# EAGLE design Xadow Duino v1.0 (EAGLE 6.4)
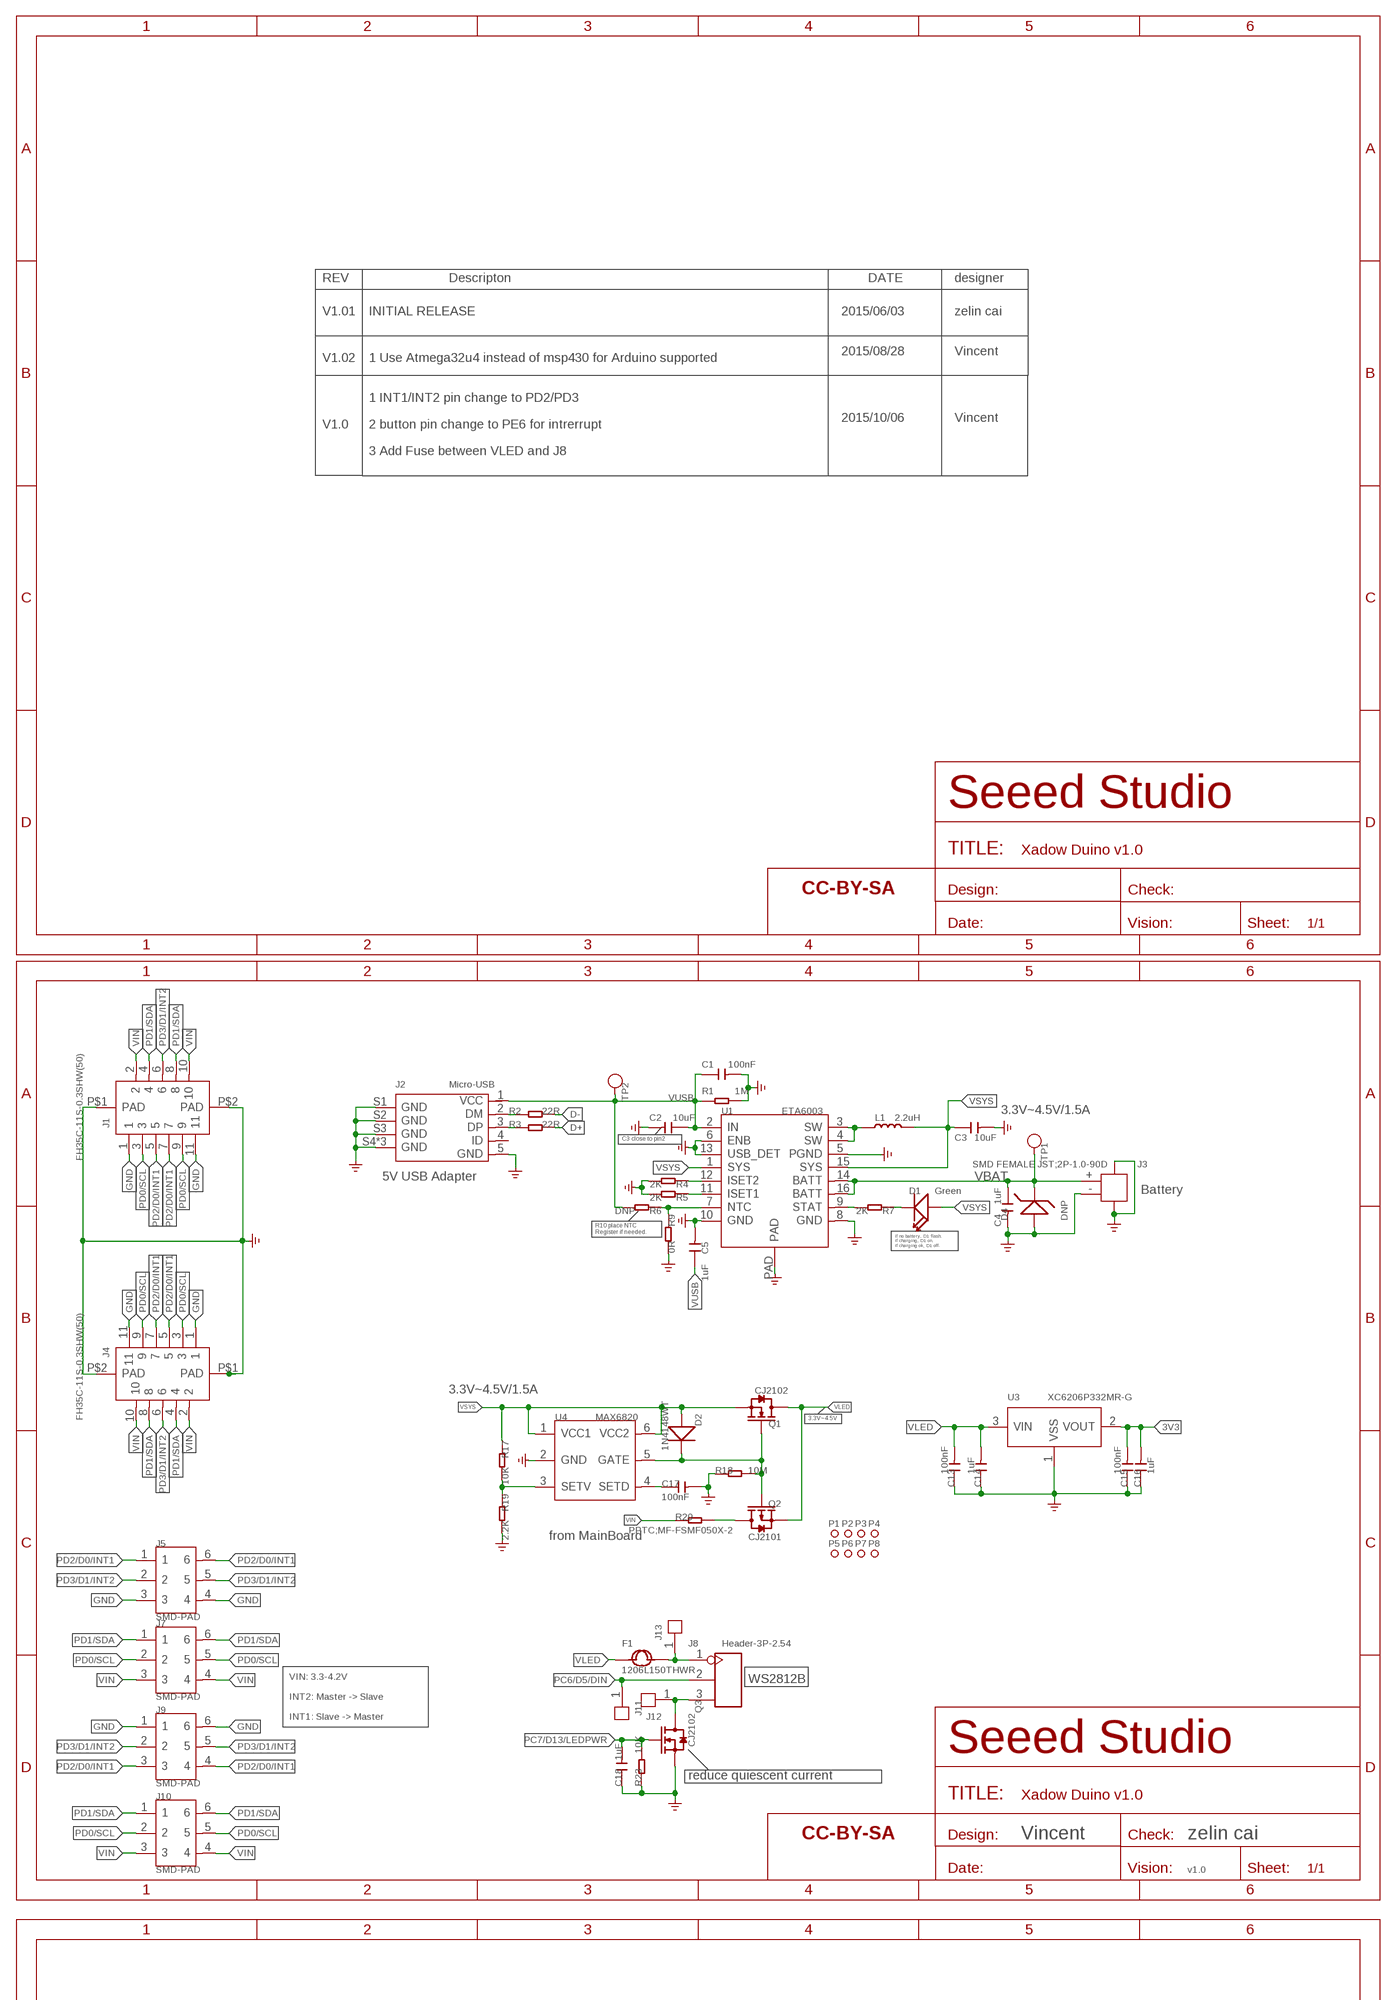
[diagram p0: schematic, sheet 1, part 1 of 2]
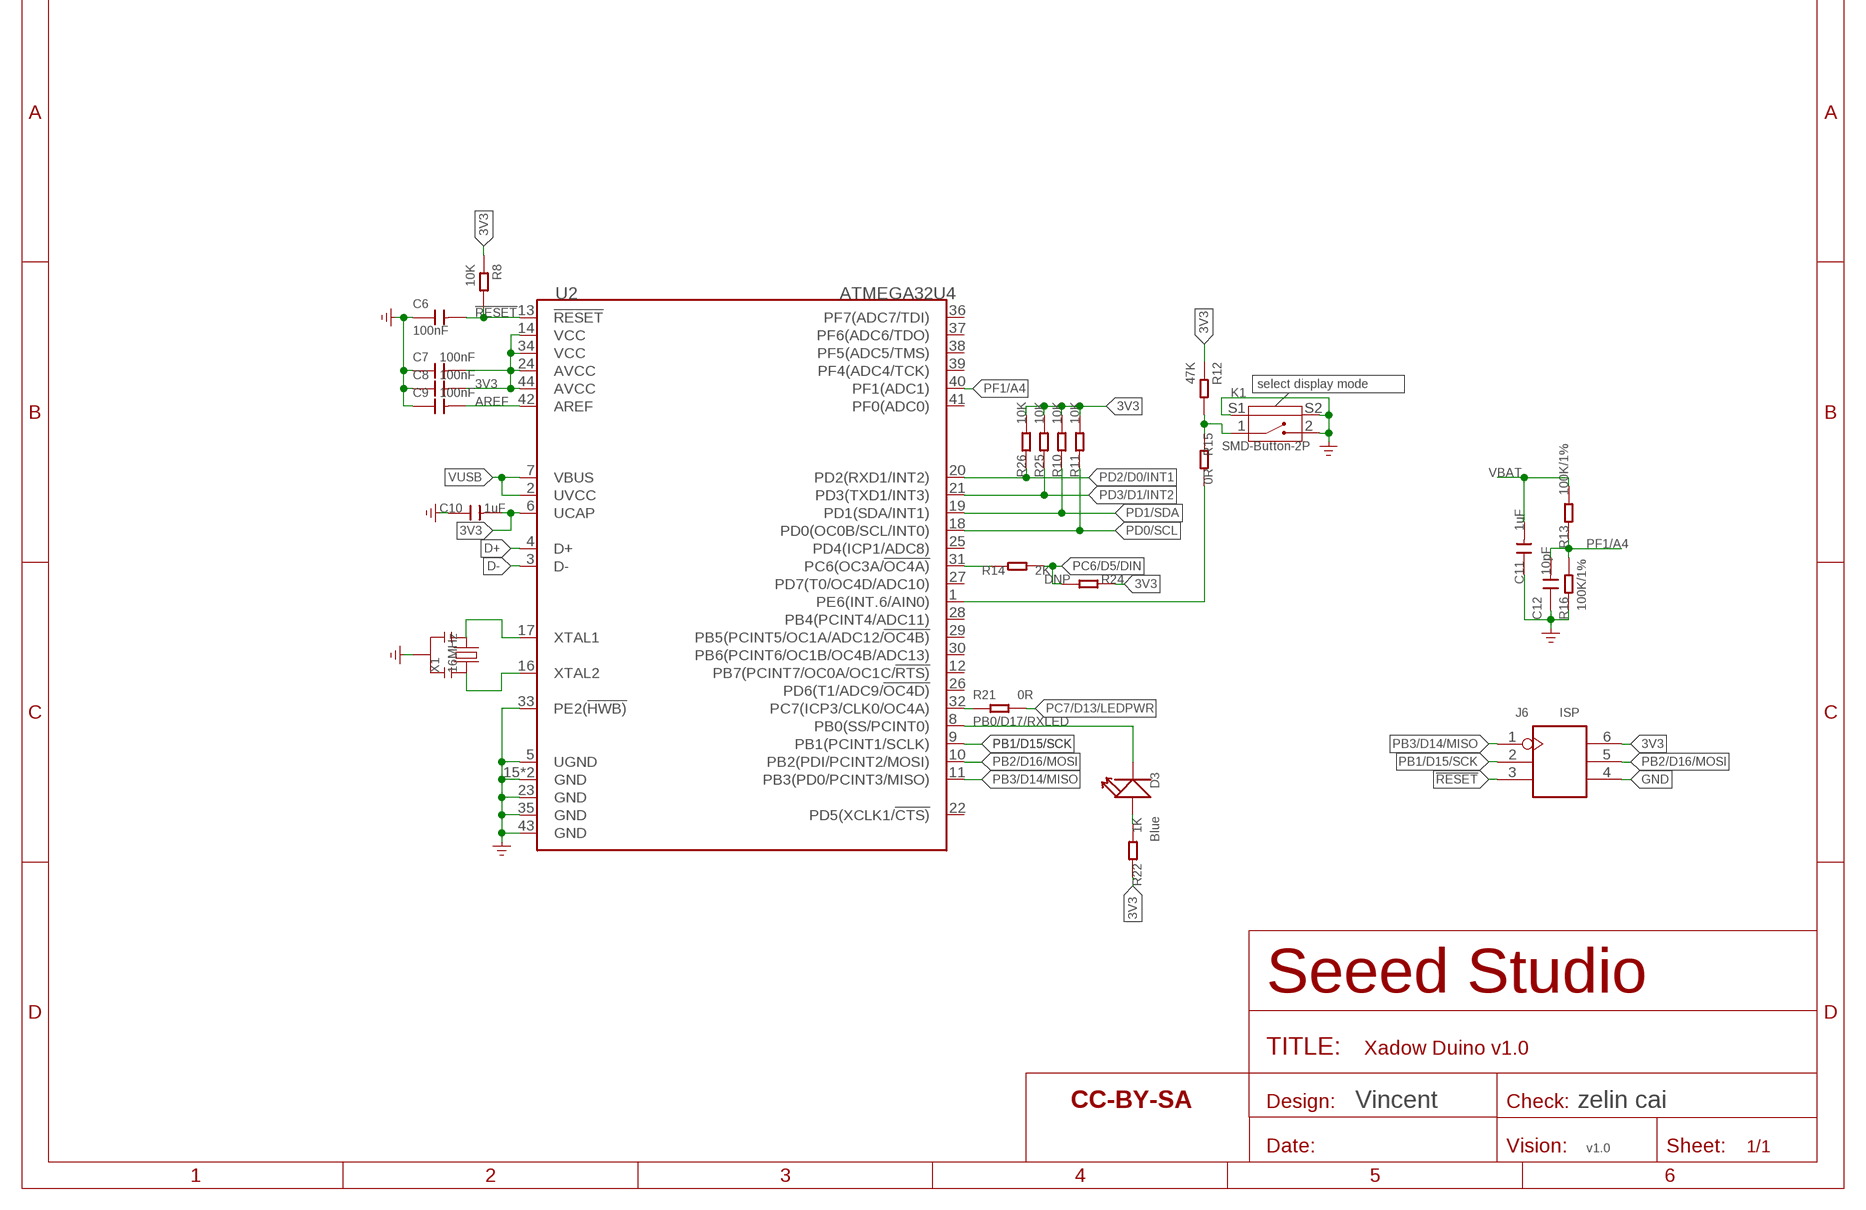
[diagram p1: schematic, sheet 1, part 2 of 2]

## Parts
C1  100nF  CAP-0201  [C0201]
C2  10uF  CAP-0603  [C0603]
C3  10uF  CAP-0603  [C0603]
C4  1uF  CAP-0402  [C0402]
C5  1uF  CAP-0402  [C0402]
C6  100nF  CAP-0201  [C0201]
C7  100nF  CAP-0201  [C0201]
C8  100nF  CAP-0201  [C0201]
C9  100nF  CAP-0201  [C0201]
C10  1uF  CAP-0402  [C0402]
C11  1uF  CAP-0402  [C0402]
C12  10pF  CAP-0201  [C0201]
C13  100nF  CAP-0201  [C0201]
C14  1uF  CAP-0402  [C0402]
C15  100nF  CAP-0201  [C0201]
C16  1uF  CAP-0402  [C0402]
C17  100nF  CAP-0201  [C0201]
C18  1uF  CAP-0402  [C0402]
D1  Green  LED'0402'  [LED-0402]
D2  1N4148WT  DIODE'0603'  [SOD-523]
D3  Blue  LED'0402'  [LED-0402]
D4  DNP  D-ZENER-2P'BZX584CX'  [SOD-523]
F1  1206L150THWR  FUSE'1206'  [F1206]
FR1  SEEEDSTUDIO-OPEN-SCH-FRAME  [SEEEDSTUDIO-PCB-FRAME]
FR2  SEEEDSTUDIO-OPEN-SCH-FRAME  [SEEEDSTUDIO-PCB-FRAME]
FR3  SEEEDSTUDIO-OPEN-SCH-FRAME  [SEEEDSTUDIO-PCB-FRAME]
J1  FH35C-11S-0.3SHW(50)  FPC-CONNECTER-11P(FH35C-11S-0.3SHW(50))  [FPC11-SMD-0.3(FH35C)]
J2  Micro-USB  MICRO-USB5+4P'5+4P'  [MICRO-USB5+4P-SMD-0.65-B]
J3  SMD FEMALE JST;2P-1.0-90D  JST-2P-SMD'1.0'  [HW2-SMD-1.0-90D]
J4  FH35C-11S-0.3SHW(50)  FPC-CONNECTER-11P(FH35C-11S-0.3SHW(50))  [FPC11-SMD-0.3(FH35C)]
J5  SMD-PAD  HEADER6_ROUND  [6P-DIP-2_ROUND]
J6  ISP  HEADER-2X3P-2.54-1.65  [H2X3P-SMD-2.54(1.65)]
J7  SMD-PAD  HEADER6  [6P-DIP-2]
J8  Header-3P-2.54  HEADER-3P-2.0  [H3-2.0]
J9  SMD-PAD  HEADER6_ROUND  [6P-DIP-2_ROUND]
J10  SMD-PAD  HEADER6  [6P-DIP-2]
J11  HEADER-1P-1.5MM  [1P-3.5/1.5MM]
J12  HEADER-1P-1.5MM  [1P-3.5/1.5MM]
J13  HEADER-1P-1.5MM  [1P-3.5/1.5MM]
K1  SMD-Button-2P  BUTTON-2+2P'HQ-TP-1100A'  [SW4-SMD-4.5X3.8X1.8MM-90D]
L1  2.2uH  INDUCTOR/FERRITE-BEAD'0805'  [L0805]
P1  MARK-1.0'ANNULAR'  [ROUND-MARK-1.0]
P2  MARK-1.0'ANNULAR'  [ROUND-MARK-1.0]
P3  MARK-1.0'ANNULAR'  [ROUND-MARK-1.0]
P4  MARK-1.0'ANNULAR'  [ROUND-MARK-1.0]
P5  MARK-1.0'ANNULAR'  [ROUND-MARK-1.0]
P6  MARK-1.0'ANNULAR'  [ROUND-MARK-1.0]
P7  MARK-1.0'ANNULAR'  [ROUND-MARK-1.0]
P8  MARK-1.0'ANNULAR'  [ROUND-MARK-1.0]
Q1  CJ2102  MOSFET-N'SI1304BDL'  [SOT-323]
Q2  CJ2101  MOSFET-P-SOT323  [SOT-323]
Q3  CJ2102  MOSFET-N'SI1304BDL'  [SOT-323]
R1  1M  RES-0201  [R0201]
R2  22R  RES-0201  [R0201]
R3  22R  RES-0201  [R0201]
R4  2K  RES-0201  [R0201]
R5  2K  RES-0201  [R0201]
R6  DNP  RES-0201  [R0201]
R7  2K  RES-0201  [R0201]
R8  10K  RES-0201  [R0201]
R9  0R  RES-0201  [R0201]
R10  10K  RES-0201  [R0201]
R11  10K  RES-0201  [R0201]
R12  47K  RES-0201  [R0201]
R13  100K/1%  RES-0201  [R0201]
R14  2K  RES-0201  [R0201]
R15  0R  RES-0201  [R0201]
R16  100K/1%  RES-0201  [R0201]
R17  10K  RES-0201  [R0201]
R18  10M  RES-0201  [R0201]
R19  2.2K  RES-0201  [R0201]
R20  PPTC;MF-FSMF050X-2  RES-0603  [R0603]
R21  0R  RES-0201  [R0201]
R22  1K  RES-0201  [R0201]
R23  10K  RES-0201  [R0201]
R24  DNP  RES-0201  [R0201]
R25  10K  RES-0201  [R0201]
R26  10K  RES-0201  [R0201]
TP1  TEST-POINT-23  [TP-D23MIL]
TP2  TEST-POINT-23  [TP-D23MIL]
U1  ETA6003  PMIC-ETA6003  [QFN16GA-0.5-3X3MM]
U2  ATMEGA32U4  MCU-ATMEGA32U4-MUR  [QFN44G-0.5-7X7MM]
U3  XC6206P332MR-G  PMIC-XC6206PMR  [SOT-23]
U4  MAX6820  PMIC-MAX6820  [SOT-23-6]
X1  16MHz  CRYSTAL-RESONATOR'SMD'  [3P-SMD-3.6X1.3]

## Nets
3V3: C7.2 C8.2 C10.2 C15.2 C16.2 J6.6 R8.1 R10.2 R11.2 R12.1 R22.1 R24.1 R25.1 R26.2 U2.6(UCAP) U2.14(VCC) U2.24(AVCC) U2.34(VCC) U2.44(AVCC) U3.2(VOUT)
!RESET: C6.2 J6.3 R8.2 U2.13(!RESET)
AREF: C9.2 U2.42(AREF)
D+: R3.2 U2.4(D+)
D-: R2.2 U2.3(D-)
GND: C1.2 C2.2 C3.2 C4.2 C5.2 C6.1 C7.1 C8.1 C9.1 C10.1 C11.1 C12.1 C13.1 C14.1 C15.1 C16.1 C17.2 C18.1 D4.+ J1.1 J1.11 J1.P$1(PAD) J1.P$2(PAD) J2.5(GND) J2.S1(GND) J2.S2(GND) J2.S3(GND) J2.S4(GND) J2.S5(GND) J2.S6(GND) J3.3 J3.4 J3.- J4.1 J4.11 J4.P$1(PAD) J4.P$2(PAD) J5.3 J5.4 J6.4 J9.1 J9.6 K1.2 K1.S1 K1.S2 Q3.2(S) R1.2 R4.2 R5.2 R9.2 R16.1 R18.1 R19.2 R23.1 U1.5(PGND) U1.6(ENB) U1.8(GND) U1.10(GND) U1.13(USB_DET) U1.PAD U2.5(UGND) U2.15(GND) U2.23(GND) U2.33(PE2(!HWB)) U2.35(GND) U2.43(GND) U2.TAB(GND) U3.1(VSS) U4.2(GND) X1.2 ; supply symbol labelled GND_POWER
N$1: Q2.3(D) R20.2
N$2: C17.1 U4.4(SETD)
N$3: D2.- Q1.1(G) Q2.1(G) R18.2 U4.5(GATE)
N$4: R15.2 U2.1(PE6(INT.6/AIN0))
N$5: R7.2 U1.9(STAT)
N$6: L1.1 U1.3(SW) U1.4(SW)
N$7: D1.- R7.1
N$8: R4.1 U1.12(ISET2)
N$9: R5.1 U1.11(ISET1)
N$11: R6.1 R9.1 U1.7(NTC)
N$12: R17.2 R19.1 U4.3(SETV)
N$13: F1.2 J8.1 J13.1
N$14: J8.3 J12.1 Q3.3(D)
N$17: J2.2(DM) R2.1
N$18: J2.3(DP) R3.1
N$19: U2.17(XTAL1) X1.1
N$20: U2.16(XTAL2) X1.3
N$21: R14.1 U2.31(PC6(OC3A/!OC4A))
N$22: R21.1 U2.32(PC7(ICP3/CLK0/OC4A))
N$23: K1.1 R12.2 R15.1
N$24: D3.+ R22.2
PB0/D17/RXLED: D3.- U2.8(PB0(SS/PCINT0))
PB1/D15/SCK: J6.2 U2.9(PB1(PCINT1/SCLK))
PB2/D16/MOSI: J6.5 U2.10(PB2(PDI/PCINT2/MOSI))
PB3/D14/MISO: J6.1 U2.11(PB3(PD0/PCINT3/MISO))
PC6/D5/DIN: J8.2 J11.1 R14.2 R24.2
PC7/D13/LEDPWR: C18.2 Q3.1(G) R21.2 R23.2
PD0/SCL: J1.3 J1.9 J4.3 J4.9 J7.2 J7.5 J10.2 J10.5 R11.1 U2.18(PD0(OC0B/SCL/INT0))
PD1/SDA: J1.4 J1.8 J4.4 J4.8 J7.1 J7.6 J10.1 J10.6 R10.1 U2.19(PD1(SDA/INT1))
PD2/D0/INT1: J1.5 J1.7 J4.5 J4.7 J5.1 J5.6 J9.3 J9.4 R26.1 U2.20(PD2(RXD1/INT2))
PD3/D1/INT2: J1.6 J4.6 J5.2 J5.5 J9.2 J9.5 R25.2 U2.21(PD3(TXD1/INT3))
PF1/A4: C12.2 R13.1 R16.2 U2.40(PF1(ADC1))
VBAT: C4.1 C11.2 D4.- J3.+ R13.2 TP1.T U1.14(BATT) U1.16(BATT)
VIN: J1.2 J1.10 J4.2 J4.10 J7.3 J7.4 J10.3 J10.4 R20.1
VLED: C13.2 C14.2 F1.1 Q1.3(D) Q2.2(S) U3.3(VIN)
VSYS: C3.1 D1.+ D2.+ L1.2 Q1.2(S) R17.1 U1.1(SYS) U1.15(SYS) U4.1(VCC1) U4.6(VCC2)
VUSB: C1.1 C2.1 C5.1 J2.1(VCC) R1.1 R6.2 TP2.T U1.2(IN) U2.2(UVCC) U2.7(VBUS)
Unconnected: J2.4(ID) U2.12(PB7(PCINT7/OC0A/OC1C/!RTS)) U2.22(PD5(XCLK1/!CTS)) U2.25(PD4(ICP1/ADC8)) U2.26(PD6(T1/ADC9/!OC4D)) U2.27(PD7(T0/OC4D/ADC10)) U2.28(PB4(PCINT4/ADC11)) U2.29(PB5(PCINT5/OC1A/ADC12/!OC4B)) U2.30(PB6(PCINT6/OC1B/OC4B/ADC13)) U2.36(PF7(ADC7/TDI)) U2.37(PF6(ADC6/TDO)) U2.38(PF5(ADC5/TMS)) U2.39(PF4(ADC4/TCK)) U2.41(PF0(ADC0))

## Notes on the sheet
- REV | Descripton | DATE | designer
- V1.01 | INITIAL RELEASE | 2015/06/03 | zelin cai
- 2015/08/28 | Vincent
- V1.02 | 1 Use Atmega32u4 instead of msp430 for Arduino supported
- 1 INT1/INT2 pin change to PD2/PD3
- 2015/10/06 | Vincent
- V1.0 | 2 button pin change to PE6 for intrerrupt
- 3 Add Fuse between VLED and J8
- 3.3V~4.5V/1.5A
- C3 close to pin2
- 5V USB Adapter
- Battery
- R10 place NTC 
  Register if needed.
- if no battery, D1 flash.
  if charging, D1 on.
  if charging ok, D1 off.
- 3.3V~4.5V/1.5A
- 3.3V~4.5V
- from MainBoard
- VIN: 3.3-4.2V
- WS2812B
- INT2: Master -> Slave
- INT1: Slave -> Master
- reduce quiescent current
- Vincent | zelin cai
- v1.0
- select display mode
- Vincent | zelin cai
- v1.0

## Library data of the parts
C1-C18 = Discrete-new:CAP: Ceramic Capacitors
D1 D3 = Discrete-new:LED
D2 = Discrete-new:DIODE*
D4 = Discrete-new:D-ZENER-2P: SOD-123:304030008;SOT-23:304030000
F1 = Discrete-new:FUSE
FR1-FR3 = moudle-new:SEEEDSTUDIO-OPEN-SCH-FRAME
J1 J4 = template:FPC-CONNECTER-11P(FH35C-11S-0.3SHW(50))
J2 = Connector-new:MICRO-USB5+4P: 5+4P-SMD-0.65-B:320010000;5+2P-SMD-0.65-AB:340032001
J3 = Connector-new:JST-2P-SMD: 2P-SMD-1.0-90D:320110054;2P-SMD-2.0-90D:320110026
J5 J9 = template:HEADER6_ROUND
J6 = Connector-new:HEADER-2X3P
J7 J10 = template:HEADER6
J8 = Connector-new:HEADER-3P
J11-J13 = Connector-new:HEADER-1P
K1 = Discrete-new:BUTTON-2+2P: SW4-SMD-4.5X3.8X1.8MM-90D:311020035;SW4-SMD-7.0X3.5X3.5MM-90D:311020023
L1 = Discrete-new:INDUCTOR/FERRITE-BEAD
P1-P8 = Discrete-new:MARK-1.0; PARTNO: DNP
Q1 Q3 = Discrete-new:MOSFET-N
Q2 = Discrete-new:MOSFET-P
R1-R26 = Discrete-new:RES
TP1 TP2 = Discrete-new:TEST-POINT
U1 = template:PMIC-ETA6003: 310990023
U2 = IC-new:MCU-ATMEGA32U4: TQFP-44:310010010;VQFN-44:310010016
U3 = IC-new:PMIC-XC6206P: LOW ESR Cap.Compatible Positive Voltage Regulators
U4 = template:PMIC-MAX6820: 310030267
X1 = Discrete:CRYSTAL-RESONATOR: Resonator Small SMD resonator. This is the itty bitty 10/20MHz resonators with built in caps. CSTCE10M0G55 and CSTCE20M0V53. Footprint has been reviewed closely but hasn't been tested yet.

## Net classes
0 default: width 0.025 mm, drill 0.203 mm, clearance 0.102 mm

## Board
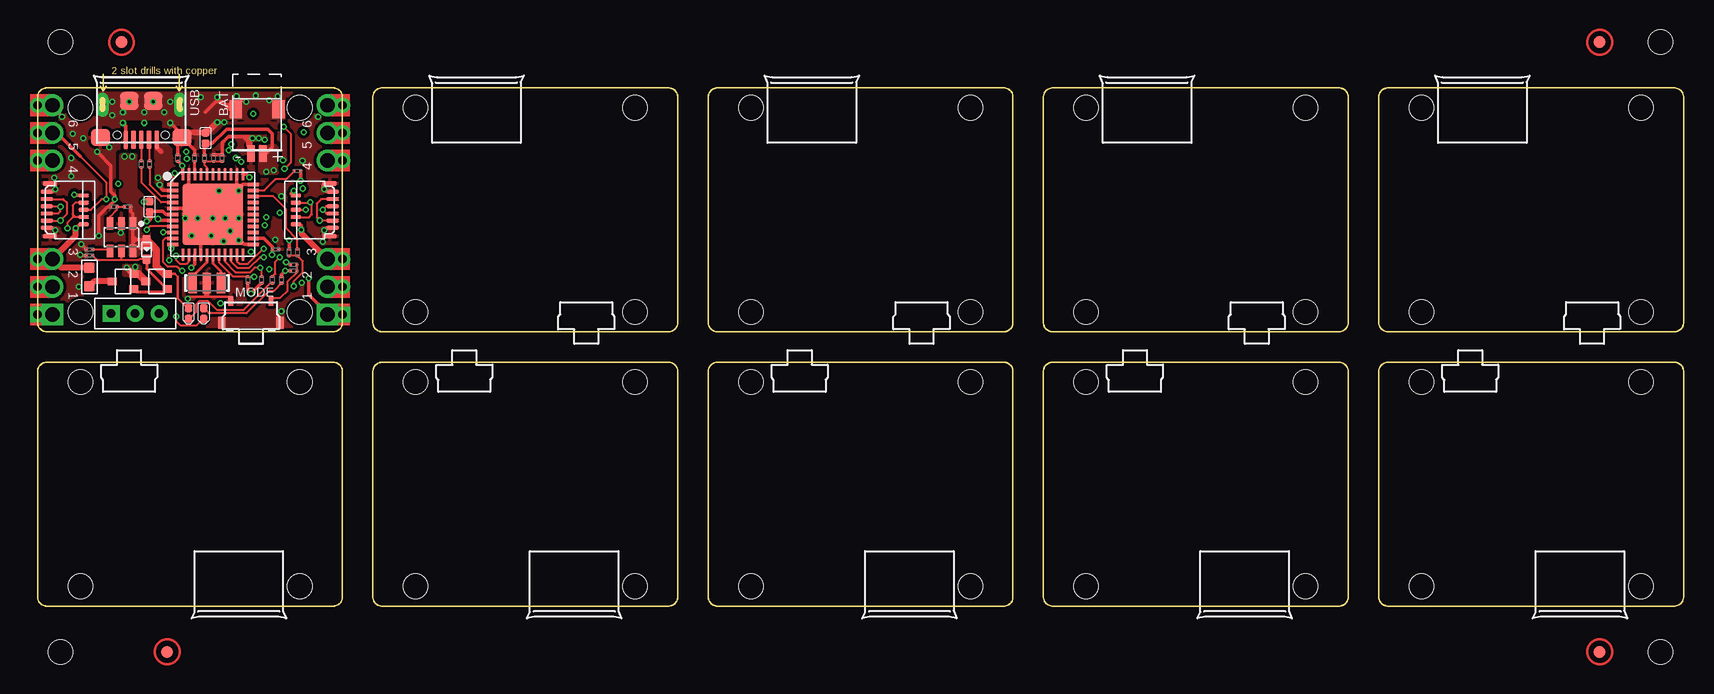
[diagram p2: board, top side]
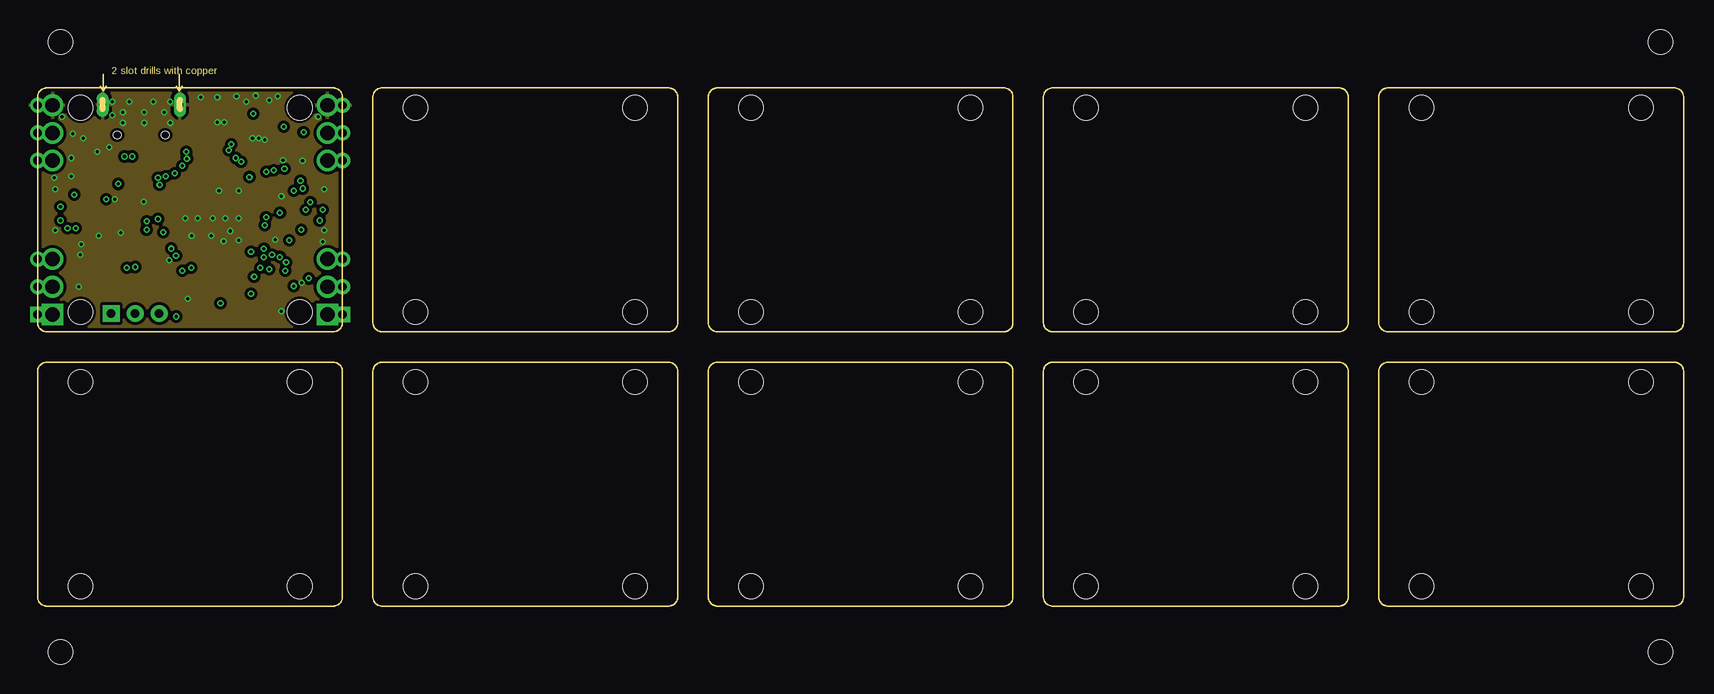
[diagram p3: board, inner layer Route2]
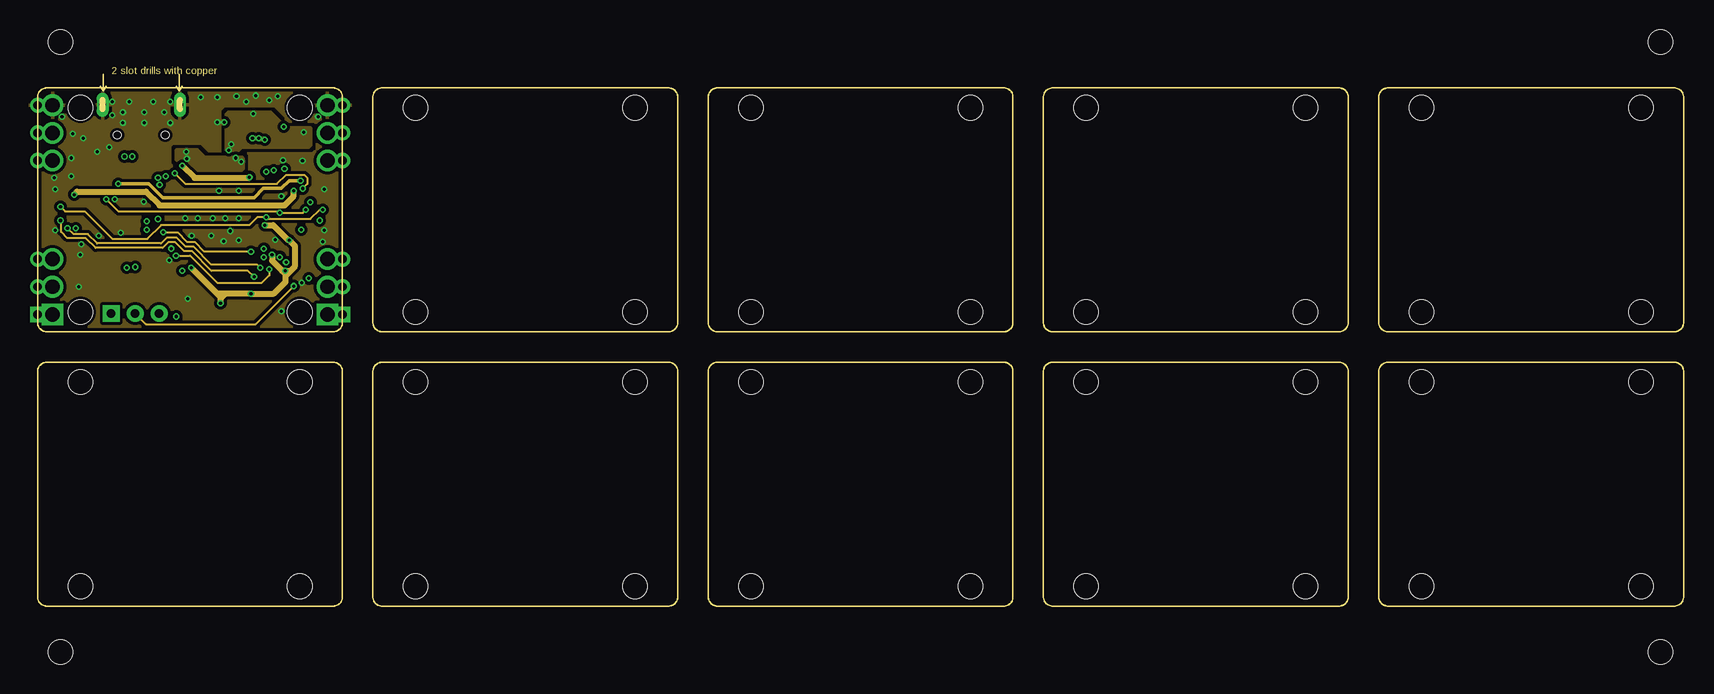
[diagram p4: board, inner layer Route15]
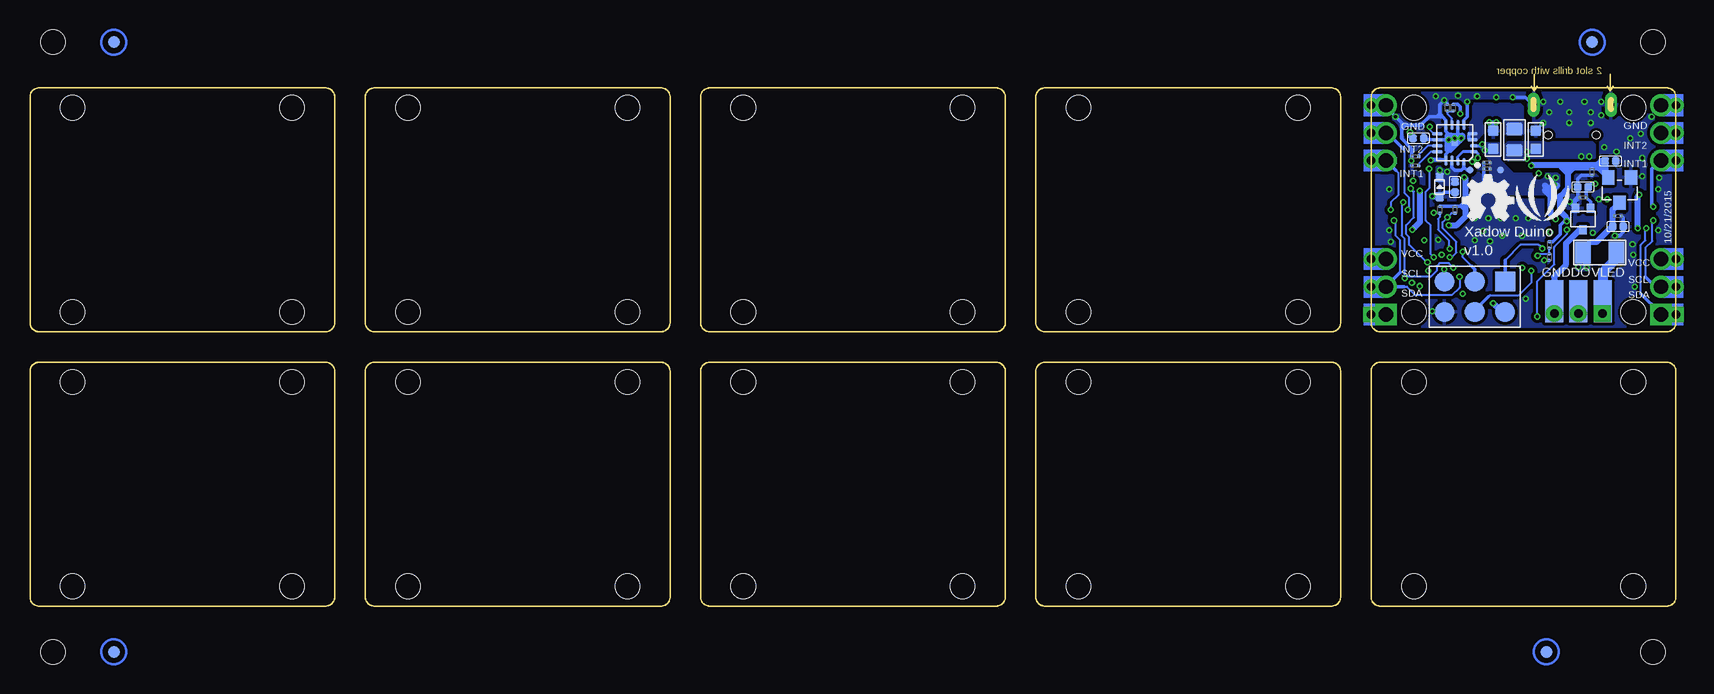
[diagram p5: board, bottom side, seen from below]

Size 137.16 x 43.18 mm. Coordinates in mm from the lower left corner, seen from the top.
Outline: 80 segments
Copper layers (1*2*15*16): Top 0.035mm / dielectric 0.2mm / Route2 0.0175mm / dielectric 0.3mm / Route15 0.0175mm / dielectric 0.2mm / Bottom 0.035mm
Design rules "SeeedStudio_4layer_DRU_no_angle_20140221 *": minimum track width 1mil, minimum drill 10mil, track to track 6mil, track to pad 6mil, pad to pad 6mil, via to via 6mil, smd to smd 0mil, copper to edge 10mil, drill to drill 8mil, minimum pad ring 6mil, minimum via ring 4mil, stop-mask expansion 4mil, vias tented up to drill 100mil, thermal gap 10mil
Holes 2.03 mm at 21.84,24.51 3.56,41.53 21.84,41.53 3.56,24.51 49.78,24.51 31.5,41.53 49.78,41.53 31.5,24.51 77.72,24.51 59.44,41.53 77.72,41.53 59.44,24.51 105.66,24.51 87.38,41.53 105.66,41.53 87.38,24.51 87.38,18.67 105.66,1.65 87.38,1.65 105.66,18.67 59.44,18.67 77.72,1.65 59.44,1.65 77.72,18.67 31.5,18.67 49.78,1.65 31.5,1.65 49.78,18.67 3.56,18.67 21.84,1.65 3.56,1.65 21.84,18.67 133.6,24.51 115.32,41.53 133.6,41.53 115.32,24.51 115.32,18.67 133.6,1.65 115.32,1.65 133.6,18.67 1.9,46.99 135.26,46.99 135.26,-3.81 1.9,-3.81
bRestrict: 1 lines

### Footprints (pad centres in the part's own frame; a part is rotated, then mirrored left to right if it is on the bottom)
C0201 = smd 0.279 x 0.318: 1 -0.279,0; 2 0.279,0
C0603 = smd 0.889 x 0.889: 1 0,0.762; 2 0,-0.762
C0402 = smd 0.635 x 0.635: 1 0,0.445; 2 0,-0.445
LED-0402 = smd 0.635 x 0.635: + -0.445,0; - 0.445,0
SOD-523 = smd 0.762 x 0.7: + -0.8,0; - 0.8,0
F1206 = smd 1.27 x 1.778: 1 -1.397,0; 2 1.397,0
FPC11-SMD-0.3(FH35C) = smd 0.3 x 1: 1 -1.5,-3.075; 3 -0.9,-3.075; 5 -0.3,-3.075; 7 0.3,-3.075; 9 0.9,-3.075; 11 1.5,-3.075 | smd 0.3 x 0.85: 2 -1.2,0; 4 -0.6,0; 6 0,0; 8 0.6,0; 10 1.2,0 | smd 0.4 x 1.15: P$1 2.2,-2.8; P$2 -2.2,-2.8
MICRO-USB5+4P-SMD-0.65-B = smd 0.381 x 1.524: 1 -1.3,-0.25; 2 -0.65,-0.25; 3 0,-0.25; 4 0.65,-0.25; 5 1.3,-0.25 | smd 1.6 x 1.397: S1 -3.4,-0.427; S6 3.4,-0.427 | drill 0.508 pad 1.016 long: S2 -3.226,-3.175; S5 3.226,-3.175 | smd 1.5 x 1.5: S3 -1,-3.5; S4 1,-3.5 | hole 0.635: -2,-0.65; 2,-0.65
HW2-SMD-1.0-90D = smd 1.524 x 1.016: 3 -3.429,1.778; 4 -3.429,-1.778 | smd 1.397 x 0.635: + 0.254,0.508; - 0.254,-0.508
6P-DIP-2_ROUND = drill 0.7 pad 1.27: 1 -2.3,0; 2 0,0; 3 2.3,0 | drill 1.2 pad 1.8: 4 2.3,1.25; 5 0,1.25; 6 -2.3,1.25
H2X3P-SMD-2.54(1.65) = smd 1.65 x 1.65: 1 -1.27,2.54; 2 -1.27,0; 3 -1.27,-2.54; 4 1.27,-2.54; 5 1.27,0; 6 1.27,2.54
6P-DIP-2 = drill 0.7 pad 1.27 square: 1 -2.3,0 | drill 0.7 pad 1.27: 2 0,0; 3 2.3,0 | drill 1.2 pad 1.8: 4 2.3,1.25; 5 0,1.25 | drill 1.2 pad 1.8 square: 6 -2.3,1.25
H3-2.0 = drill 0.7 pad 1.4 square: 1 0,2 | drill 0.7 pad 1.4: 2 0,0; 3 0,-2
1P-3.5/1.5MM = smd 1.5 x 3.5: 1 0,0
SW4-SMD-4.5X3.8X1.8MM-90D = smd 0.4 x 0.8: 1 -1.675,-1.277; 2 1.675,-1.277 | smd 0.6 x 1: S1 -2.425,0.5; S2 2.425,0.5
L0805 = smd 1.016 x 1.397: 1 -0.889,0; 2 0.889,0
ROUND-MARK-1.0 = smd 1.016 x 1.016: P$1 0,0
SOT-323 = smd 0.635 x 0.762: 1 -0.635,-0.889; 2 0.635,-0.889; 3 0,0.889
R0201 = smd 0.279 x 0.318: 1 -0.279,0; 2 0.279,0
R0603 = smd 0.889 x 0.889: 1 0,0.762; 2 0,-0.762
TP-D23MIL = smd 0.6 x 0.6: T 0,0
QFN16GA-0.5-3X3MM = smd 0.65 x 0.28: 1 -1.575,0.75; 2 -1.575,0.25 | smd 0.85 x 0.28: 3 -1.475,-0.25; 4 -1.475,-0.75; 9 1.475,-0.75; 10 1.475,-0.25; 11 1.475,0.25; 12 1.475,0.75 | smd 0.28 x 0.85: 5 -0.75,-1.475; 6 -0.25,-1.475; 7 0.25,-1.475; 8 0.75,-1.475; 13 0.75,1.475; 14 0.25,1.475 | smd 0.28 x 0.65: 15 -0.25,1.575; 16 -0.75,1.575 | smd 0.508 x 0.508: PAD 0,0
QFN44G-0.5-7X7MM = smd 1 x 0.3: 1 -3.35,2.5; 2 -3.35,2; 3 -3.35,1.5; 4 -3.35,1; 5 -3.35,0.5; 6 -3.35,0; 7 -3.35,-0.5; 8 -3.35,-1; 9 -3.35,-1.5; 10 -3.35,-2; 11 -3.35,-2.5; 23 3.35,-2.5; 24 3.35,-2; 25 3.35,-1.5; 26 3.35,-1; 27 3.35,-0.5; 28 3.35,0; 29 3.35,0.5; 30 3.35,1; 31 3.35,1.5; 32 3.35,2; 33 3.35,2.5 | smd 0.3 x 1: 12 -2.5,-3.35; 13 -2,-3.35; 14 -1.5,-3.35; 15 -1,-3.35; 16 -0.5,-3.35; 17 0,-3.35; 18 0.5,-3.35; 19 1,-3.35; 20 1.5,-3.35; 21 2,-3.35; 22 2.5,-3.35; 34 2.5,3.35; 35 2,3.35; 36 1.5,3.35; 37 1,3.35; 38 0.5,3.35; 39 0,3.35; 40 -0.5,3.35; 41 -1,3.35; 42 -1.5,3.35; 43 -2,3.35; 44 -2.5,3.35 | smd 5.08 x 5.08: TAB 0,0
SOT-23 = smd 1.016 x 1.2: 1 -0.95,-1.06; 2 0.95,-1.06; 3 0,1.06
SOT-23-6 = smd 0.55 x 1.016: 1 -0.95,-1.143; 2 0,-1.143; 3 0.95,-1.143; 4 0.95,1.143; 5 0,1.143; 6 -0.95,1.143
3P-SMD-3.6X1.3 = smd 0.7 x 1.7: 1 -1.2,0; 2 0,0; 3 1.2,0

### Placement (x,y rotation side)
C1  15.75,36.96 180 bottom
C2  15.24,38.86 180 bottom
C3  11.68,38.86 180 bottom
C4  18.42,34.92 0 bottom
C5  21.46,38.99 90 bottom
C6  10.54,29.08 90 bottom
C7  19.81,29.72 180 top
C8  11.68,37.34 270 top
C9  13.08,37.34 270 top
C10  9.33,33.27 0 top
C11  13.99,39 0 top
C12  14.67,37.34 270 top
C13  4.83,32.51 180 bottom
C14  4.83,31.62 270 bottom
C15  6.99,36.2 90 bottom
C16  5.46,37.08 270 bottom
C17  4.32,29.72 180 top
C18  7.75,34.92 90 bottom
D1  12.57,24.38 270 top
D2  9.08,29.72 270 top
D3  13.84,24.38 270 top
D4  19.68,34.92 90 bottom
F1  6.35,29.46 0 bottom
FR1  not placed on the board
FR2  not placed on the board
FR3  not placed on the board
J1  21.53,33.02 90 top
J2  8.64,38.61 180 top
J3  18.29,37.97 270 top
J4  3.84,33.02 270 top
J5  25.4,39.43 90 top
J6  16.76,25.78 270 bottom
J7  25.4,26.61 90 top
J8  8.13,24.38 90 top
J9  0,39.43 270 top
J10  0,26.61 90 bottom
J11  8.13,25.4 0 bottom
J12  10.16,25.4 0 bottom
J13  6.1,25.4 0 bottom
K1  17.78,24.13 180 top
L1  13.46,38.86 270 bottom
P1  not placed on the board
P2  not placed on the board
P3  not placed on the board
P4  not placed on the board
P5  not placed on the board
P6  not placed on the board
P7  not placed on the board
P8  not placed on the board
Q1  9.91,27.05 90 top
Q2  7.11,27.05 90 top
Q3  7.75,32.26 180 bottom
R1  15.75,36.45 180 bottom
R2  9.33,36.83 270 top
R3  8.64,36.83 270 top
R4  21.72,36.7 180 bottom
R5  21.72,37.47 180 bottom
R6  18.55,41.53 90 bottom
R7  19.56,27.18 90 top
R8  10.54,30.1 270 bottom
R9  19.05,41.53 90 bottom
R10  18.67,27.18 270 top
R11  17.53,27.18 270 top
R12  21.34,27.94 0 top
R13  13.91,37.34 90 top
R14  21.65,29.46 270 top
R15  21.34,28.45 180 top
R16  15.37,37.34 270 top
R17  7.49,33.27 180 top
R18  4.32,29.21 0 top
R19  6.35,33.27 180 top
R20  4.32,27.43 0 top
R21  21.65,36.26 0 top
R22  20.32,27.18 270 top
R23  7.75,34.04 0 bottom
R24  20.96,29.46 270 top
R25  19.68,33.02 270 bottom
R26  18.42,33.02 90 bottom
TP1  17.14,36.32 0 bottom
TP2  14.61,36.32 0 bottom
U1  18.42,38.61 180 bottom
U2  14.61,32.64 0 top
U3  4.7,34.67 180 bottom
U4  6.99,30.73 180 top
U$1  [OSHW_FILLX150_NOTEXT]  17.78,32.13 0 bottom
U$3  [SEEED-LOGO-150]  13.33,32.13 0 bottom
X1  14.1,26.92 180 top

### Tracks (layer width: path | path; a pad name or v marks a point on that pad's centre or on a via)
3V3  (via drill 0.25 pad 0.51)
  Top 0.254: C8.2 11.71,37.06
  Top 0.305: C10.2 9.4,32.89 10.41,32.89 10.67,32.64 U2.6 | U2.14 13.11,28.5 v12.8,28.19 | U2.34 17.41,35.99 v17.65,35.75 | U2.44 12.11,36.66 v12.07,36.7 11.71,37.06 | U2.24 18.85,30.64 19.53,29.96 C7.2 v19.53,29.29 | R11.2 17.53,26.29 v17.78,26.04 18.64,26.9 R10.2 | R22.1 20.32,27.62 v20.64,27.94 R12.1 | R24.1 20.96,30.48 v20.96,30.49
  Top 0.508: C10.2 9.33,32.32 v9.09,32.08
  Route15 0.305: v20.96,30.49 20.96,30.47 21.21,30.23
  Route15 0.508: v12.07,36.7 13.08,35.69 17.59,35.69 v17.65,35.75 | 15.62,26.04 v17.78,26.04 19.68,26.04 20.64,26.99 20.64,27.5 | 15.62,26.04 15.24,26.04 | 15.24,26.04 14.96,26.04 | 14.96,26.04 v12.8,28.19 | v15.24,25.23 15.24,25.65 | 15.24,25.76 15.24,26.04 | 15.24,25.65 15.24,25.76 | 15.24,25.76 14.96,26.04 | 15.24,25.65 15.62,26.04 | v19.53,29.29 19.53,28.79 20.38,27.94 | v20.64,27.94 20.38,27.94 | v20.64,27.94 20.64,27.5 | v20.64,27.94 21.08,27.94 | 21.08,27.94 21.46,28.32 21.46,29.99 v20.96,30.49 20.88,30.49 19.63,31.74 v18.92,31.74 | 20.64,27.5 21.08,27.94 | 20.38,27.94 20.7,27.62
  Bottom 0.305: R8.1 10.26,30.38 9.65,30.99 9.65,31.75 9.32,32.08 9.14,32.08 | 9.08,32.07 v9.09,32.08 9.14,32.08 | 8.99,32.23 9.14,32.08 | 9.02,32 9.14,32.13 | C15.2 6.83,36.47 6.73,36.58 | 18.01,33.3 R26.2 R25.1 | 17.93,33.3 17.55,33.3 17.53,33.27 | 18.01,33.3 17.65,33.66 | 18.01,33.3 17.93,33.3 | 17.93,33.3 17.65,33.02
  Bottom 0.508: v17.65,35.75 17.53,35.62 17.53,33.27 17.53,32.47 18.26,31.74 v18.92,31.74 | 9.02,36.58 9.02,36.07 | 9.02,36.07 9.02,34.8 9.65,34.16 9.65,32.89 9.14,32.38 9.14,32.13 9.14,32.08 | J6.6 14.52,24.51 v15.24,25.23 | 6.48,36.83 6.22,37.08 C16.2 5.91,35.86 5.78,35.86 U3.2 | 6.54,36.77 6.73,36.58 | 6.48,36.83 6.41,36.77 | 6.41,36.77 5.97,36.32 | 6.48,36.58 6.1,36.58 | 9.02,36.58 9.53,36.58 9.02,36.07 | 9.02,36.58 8.51,36.58 | 8.51,36.58 6.73,36.58 | 9.02,36.07 8.51,36.58 | 6.73,36.58 6.48,36.58 | 6.48,36.58 5.97,36.07 | 6.48,36.7 6.41,36.77 | v12.07,36.7 12,36.77 6.54,36.77 | 6.54,36.77 6.48,36.83
!RESET  (via drill 0.25 pad 0.51)
  Top 0.152: U2.13 12.61,28.72 12.39,28.5 11.89,28.5 11.53,28.85 v11.53,29.2
  Route15 0.152: v11.53,29.2 12.71,29.2 14.99,26.92 18.67,26.92 19.3,27.56 v19.3,28.07
  Bottom 0.152: v11.53,29.21 v11.53,29.2 11.42,29.31 10.67,29.31 10.62,29.36 C6.2 R8.2 | 19.3,27.81 v19.3,28.07
  Bottom 0.305: J6.3 19.3,27.81
AREF
  Top 0.254: U2.42 13.11,37.03 C9.2
D+
  Top 0.152: U2.4 10.3,33.64 8.64,35.31 R3.2
D-
  Top 0.152: R2.2 9.33,35.12 10.31,34.14 U2.3
GND  (via drill 0.25 pad 0.51)
  Top 0.203: X1.2 14.1,26.04 | 14.1,26.04 14.22,25.91 | 14.22,25.91 14.35,25.78 | 14.35,25.78 15.87,25.78 16.11,25.55 K1.2 | 14.35,25.78 12.69,25.78 v12.52,25.62 | 14.1,26.04 13.97,25.91 | 13.97,25.91 13.87,25.81 14,25.81 14.1,25.91 | 13.97,25.91 13.97,26.29 | 14.22,25.91 14.22,26.29
  Top 0.305: U2.5 12.07,33.14 12.32,32.89 v12.32,32.32 12.32,31.38 v12.83,30.87 | J4.P$1 1.29,30.82 1.52,31.05 1.52,31.24 v1.46,31.3 1.25,31.52 J4.11 | J4.1 1.25,34.52 v1.46,34.73 1.52,34.8 1.52,34.99 1.29,35.22 J4.P$2 | J9.6 1.25,41.55 v2.03,40.77 | J1.P$2 24.04,30.82 23.81,31.05 23.81,31.24 v23.88,31.3 24.09,31.52 J1.1 | J1.11 24.09,34.52 v23.88,34.73 23.75,34.86 23.75,35.05 23.92,35.22 J1.P$1 | J3.3 19.81,41.4 | 16.51,41.66 J3.4 16,41.4 15.75,41.66 | 16.51,41.66 17.02,42.16 17.27,42.16 v17.4,42.04 | 15.75,41.66 15.62,41.78 | J2.S1 12.04,39.27 v11.05,40.26 | 12.07,39 13.08,37.99 C9.1 | 12.07,39 J2.S1 | U2.33 17.11,35.14 16.76,34.8 v16.76,34.61 16.73,34.64 16.61,34.64 U2.35 | U2.TAB v14.61,32.32 | U2.23 17.23,30.14 16.45,30.92 14.48,30.92 | U2.15 13.61,30.24 14.29,30.92 14.48,30.92 | U2.43 12.61,34.77 12.95,34.42 14.92,34.42 v15.11,34.61 | 17.65,39.12 15.87,39.12 15.37,38.61 R16.1 C12.1 | 17.65,39.12 17.78,39.12 v17.91,38.99 17.78,38.86 J3.- 17.78,38.1 17.53,38.35 17.53,38.73 | 17.53,38.73 17.53,38.99 17.65,39.12 | 17.53,38.73 17.27,38.99 | 12.14,39.14 J2.S1 | 15.75,41.66 16.51,41.66 | 15.62,41.78 15.95,41.78 | 15.95,41.78 16.51,41.78 | 15.95,41.78 16.15,41.99 | 13.97,41.15 14.86,42.04 | 15.62,41.78 15.37,42.04 15.24,42.04 | 14.86,42.04 15.24,42.04 | 14.86,42.04 14.99,42.16 v14.99,42.42 14.99,42.29 15.24,42.04 | C8.1 11.68,38.61 12,38.93 12.07,39 | U4.2 6.99,31.18 v6.92,31.12 | J2.5 7.34,40.03 v7.11,40.26 | C17.2 4.04,29.74 v3.62,30.16 | R18.1 3.62,29.21 v3.56,29.27 | 14.48,30.92 v14.48,30.87 | v5.08,30.86 5.08,32.51 5.84,33.27 R19.2 6.07,33.44 6.41,33.78 v6.41,33.91 6.41,34.23 6.1,34.54 6.1,36.7 v4.95,37.85
  Top 0.508: C10.1 8.86,33.72 v8.84,33.69 | 12,38.93 12.52,39.44 C11.1 14.11,39.44 v14.99,40.32
  Bottom 0.254: U1.10 20.89,38.86 C5.2
  Bottom 0.305: U1.10 18.55,38.86 v18.42,38.99 | 19.43,40.77 19.17,40.5 U1.8 19.17,39.55 18.92,39.31 18.73,39.31 v18.42,38.99 | 19.43,40.77 19.68,41.02 | C3.2 v11.05,40.26 | J5.4 24.15,41.55 v23.37,40.77 22.86,40.26 | 18.86,39.05 18.86,37.97 19.17,37.67 U1.13 19.24,37.21 20.38,37.21 v20.45,37.15 | R1.2 C1.2 16.03,35.39 | C4.2 19.33,34.48 D4.+ | C6.1 10.97,28.8 v10.99,28.82 | U1.6 18.17,39.45 | 18.17,39.45 18.17,39.24 v18.42,38.99 | 18.14,39.42 18.17,39.45 | 22.73,40.13 22.76,40.16 | 22.76,40.16 22.86,40.26 | 19.68,41.02 19.68,41.78 v19.3,42.16 19.05,41.91 R9.2 | U1.5 17.67,40.5 17.4,40.77 v17.4,42.04 | R5.2 22,38.06 22.86,38.93 22.86,39.75 | R4.2 22,37.03 v22.07,37.11 | v15.56,40.32 v14.99,40.32 15.24,40.07 C2.2 15.24,40 15.49,40.26 | 15.49,40.26 v15.56,40.32 | v15.56,40.32 15.62,40.26 15.49,40.26 | v13.59,42.42 12.57,42.42 11.94,41.78 | R23.1 8.19,34.2 C18.1 8.19,35.62 7.9,35.92 C15.1 | 8.89,33.66 Q3.2 8.38,33.68 R23.1 | v5.08,30.86 4.7,30.86 4.38,31.18 C14.1 4.38,32.35 C13.1 | R23.1 8.25,34.04 8.64,33.66 8.8,33.66 v8.84,33.69 | 19.94,40.77 20.57,40.77 21.27,40.07 22.54,40.07 | 19.94,40.77 19.43,40.77 | 22.86,39.75 22.86,40.26 | 19.68,41.02 19.94,40.77 | 22.54,40.07 22.73,40.07 22.8,40.13 22.76,40.16 | 22.54,40.07 22.86,39.75
  Bottom 0.508: D4.+ 20.28,34.12 v20.32,34.16
  other vias: 5.97,38.23 7.62,42.04 9.65,42.04 11.05,42.04 6.22,42.04 20.32,24.57 16.76,32.32 19.81,30.54 22,26.94 23.77,30.37 3.81,38.99 2.79,35.81 8.89,40.26 1.4,35.69 3.43,26.61 18.92,38.86 16.57,42.48 20,42.48 16.07,31.25 16.76,30.49 7.11,41.15 8.89,41.15 10.54,41.15 18.16,42.55 6.22,40.89 2.92,39.37 2.79,37.34 13.33,32.32 15.62,32.32 15.49,30.42
  pour Top (isolate 0.254, rank 6): -0.64,43.81 26.04,43.81 26.04,22.22 -0.64,22.22
  pour Route2 (isolate 0.254, rank 6): -0.64,43.81 26.04,43.81 26.04,22.22 -0.64,22.22
  pour Route15 (isolate 0.254, rank 6): -0.64,43.81 26.04,43.81 26.04,22.22 -0.64,22.22
  pour Bottom (isolate 0.254, rank 6): -0.64,43.81 26.04,43.81 26.04,22.22 -0.64,22.22
  pour Top (isolate 0.254, no thermals): 14.48,22.86 14.48,24.64 20.57,24.64 20.57,22.86
  pour Top (isolate 0.254, no thermals): 4.95,40.64 20.57,40.64 20.57,43.05 4.95,43.05
N$1
  Top 0.508: Q2.3 4.7,27.05 R20.2
N$2
  Top 0.152: C17.1 5.91,29.72 U4.4
N$3
  Top 0.152: D2.- 8.47,28.92 8.38,28.83 7.11,28.83 | R18.2 4.98,28.83 6.86,28.83 | 7.11,28.83 6.99,28.83 | 6.99,28.83 6.86,28.83 | U4.5 6.99,28.96 | 6.99,28.96 6.99,28.83 | 6.99,28.96 6.86,28.83 | 6.99,28.96 7.11,28.83
  Top 0.254: Q1.1 10.67,26.42 | 10.67,26.42 10.41,26.16 8.25,26.16 Q2.1 | 10.67,26.42 10.67,26.54 9.08,28.13 D2.-
N$4  (via drill 0.25 pad 0.51)
  Top 0.152: U2.1 11.26,35.89 v11.43,36.07 | R15.2 20.89,28.45 v20.7,28.64
  Route15 0.152: v11.43,36.07 12.32,35.18 19.94,35.18 20.7,35.94 22.22,35.94 22.48,35.69 22.48,35.18 v22.1,34.8
  Bottom 0.152: v20.7,28.64 20.76,28.64 22.22,30.1 22.22,30.73 22.48,30.99 22.48,31.75 21.84,32.38 21.84,34.54 v22.1,34.8
N$5  (via drill 0.25 pad 0.51)
  Top 0.152: R7.2 19.58,27.46 19.81,27.69 19.81,28.7 v20.19,29.08 | v20.57,36.45 21.08,36.96 21.08,39.37 v20.51,39.94
  Bottom 0.152: U1.9 20.18,39.36 20.51,39.69 v20.51,39.94 | v20.19,29.08 20.45,29.34 20.45,31.75 20.83,32.13 20.83,34.54 20.57,34.8 v20.57,36.45
N$6
  Bottom 0.305: U1.3 17.14,38.86 17.25,38.96 17.25,39.22 17.11,39.36 U1.4
  pour Bottom (isolate 0.254, no thermals): 14.1,39.24 12.83,39.24 12.7,39.37 12.7,41.63 12.98,41.91 16.87,41.91 17.27,41.51 17.27,38.91 17.09,38.73 16.65,38.73 16,39.38 16,40.26 15.87,40.39 14.61,40.39 14.35,40.13 14.35,39.5
N$7
  Top 0.152: D1.- 12.64,23.94 13.21,24.51 13.21,25.15 13.46,25.4 14.22,25.4 14.93,24.69 17.2,24.69 19.41,26.9 R7.1
N$8
  Bottom 0.152: U1.12 20.43,37.86 21.44,36.85 R4.1
N$9
  Bottom 0.152: U1.11 20.7,38.36 21.44,37.62 R5.1
N$11
  Bottom 0.152: U1.7 18.67,40.64 19.05,41.02 R9.1 R6.1
N$12
  Top 0.152: R17.2 R19.1 6.6,33.25 6.6,33.02 6.04,32.45 U4.3
N$13
  Bottom 0.508: J13.1 6.1,24.42 J8.1
  Bottom 0.813: F1.2 4.95,28.96 6.1,27.81 J13.1
N$14
  Bottom 0.508: J8.3 10.16,24.38 J12.1 10.16,27.43 9.14,28.45 9.14,30.23 8,31.37 Q3.3
N$17
  Top 0.152: J2.2 9.29,37.16 R2.1
N$18
  Top 0.152: J2.3 R3.1
N$19
  Top 0.254: U2.17 14.61,28.55 15.3,27.86 X1.1
N$20
  Top 0.254: U2.16 14.11,28.64 12.9,27.43 X1.3
N$21
  Top 0.152: U2.31 19.64,34.14 20.7,33.08 20.7,31.5 21.65,30.54 R14.1
N$22
  Top 0.152: U2.32 18.89,34.64 19.81,35.56 20.7,35.56 21.37,36.23 R21.1
N$23
  Top 0.152: K1.1 19.46,25.68 20.22,25.68 20.83,26.29 20.83,27.05 21.61,27.84 R12.2 R15.1
N$24
  Top 0.152: D3.+ 14.29,24.38 17.4,24.38 19.3,26.29 19.71,26.29 R22.2
PB0/D17/RXLED  (via drill 0.25 pad 0.51)
  Top 0.152: D3.- 13.78,23.94 13.21,23.37 11.94,23.37 11.56,23.75 v11.56,24.13 | U2.8 9.35,31.64 v9.08,31.37
  Bottom 0.152: v11.56,24.13 11.56,27.05 10.14,28.47 10.14,29.93 9.08,30.99 v9.08,31.37
PB1/D15/SCK  (via drill 0.25 pad 0.51)
  Top 0.152: U2.9 v10.46,31.14
  Route15 0.152: v10.46,31.14 11.66,31.14 12.45,30.35 13.08,30.35 13.91,29.53 v17.78,29.53
  Bottom 0.152: 17.02,28.32 17.78,29.08 v17.78,29.53
  Bottom 0.305: J6.2 16.76,28.07 17.02,28.32
PB2/D16/MOSI  (via drill 0.25 pad 0.51)
  Top 0.152: v12.07,27.94 11.94,27.94 11.62,28.26 10.86,28.26 10.44,28.68 10.44,30.45 10.63,30.64 U2.10
  Bottom 0.152: 15.62,25.78 15.49,25.91 13.08,25.91 12.07,26.92 v12.07,27.94
  Bottom 0.305: J6.5 16.76,24.64 15.62,25.78
PB3/D14/MISO  (via drill 0.25 pad 0.51)
  Top 0.152: U2.11 11.26,29.91 v11.14,29.79
  Bottom 0.152: v11.14,29.79 11.44,30.1 12.95,30.1 14.22,28.83
  Bottom 0.305: J6.1 14.22,28.83
PC6/D5/DIN  (via drill 0.25 pad 0.51)
  Top 0.152: v21.34,26.67 21.34,27.05 22.1,27.81 22.1,28.74 R14.2 R24.2
  Route15 0.152: v21.34,26.67 18.16,23.5 9.02,23.5 J8.2
  Bottom 0.152: J11.1 J8.2
PC7/D13/LEDPWR  (via drill 0.25 pad 0.51)
  Top 0.305: R21.2 21.93,35.46 v21.91,35.43
  Route15 0.305: v6.73,35.18 9.27,35.18 10.41,34.04 18.03,34.04 18.8,34.8 20.32,34.8 20.96,35.43 v21.91,35.43
  Bottom 0.305: Q3.1 7.11,33.68 R23.2 7.47,34.76 C18.2 7.05,35.18 v6.73,35.18
PD0/SCL  (via drill 0.25 pad 0.51)
  Top 0.152: U2.18 15.11,28.65 16.26,27.5 17.49,27.5 R11.1 18.01,27.46 v18.03,27.43 | J4.3 2.15,33.92 2.41,33.66 2.41,32.64 v1.9,32.13 v1.89,32.12 J4.9 | J1.9 23.63,33.92 23.24,33.53 23.24,32.38 v23.5,32.13 v23.51,32.12 J1.3 | J10.5 J10.2
  Route15 0.152: v1.9,32.13 1.97,32.07 1.97,31.18 2.48,30.67 4,30.67 4.83,29.84 10.41,29.84 10.92,30.35 11.43,30.35 12.19,29.59 12.83,29.59 14.48,27.94 17.53,27.94 v18.03,27.43
  Bottom 0.152: 2.54,27.43 2.54,29.84 1.97,30.42 1.97,32.07 v1.9,32.13 | 24.13,26.67 24.15,26.65 J7.5 J7.2 | 22.99,27.81 22.99,30.48 23.37,30.86 23.37,32 v23.5,32.13 | 22.63,26.61 22.63,26.62 22.43,26.62 21.72,25.91 18.67,25.91 18.03,26.54 v18.03,27.43
  Bottom 0.305: J10.5 1.71,26.61 2.54,27.43 | 22.63,26.62 24.08,26.62 24.13,26.67 22.99,27.81
PD1/SDA  (via drill 0.25 pad 0.51)
  Top 0.152: J4.4 3.14,33.62 2.92,33.4 2.92,32.66 | J4.8 2.96,32.42 2.92,32.38 | 24.08,24.31 J7.6 J7.1 | J1.4 22.64,32.42 22.86,32.64 22.86,33.53 v22.73,33.66 22.7,33.62 J1.8 | 2.92,32.38 2.49,31.95 v2.49,31.5 | 2.92,32.66 2.92,32.38 | 2.92,32.66 3.15,32.44 | J10.6 J10.1 | U2.19 15.61,28.72 16.49,27.84 17.73,27.84 18.08,28.19 v18.54,28.19 18.67,28.07 R10.1
  Top 0.305: 24.08,24.31 24.08,24.48 22.61,25.96 v22.61,27.3
  Route15 0.152: v2.49,31.5 3,30.99 4.19,30.99 4.95,30.23 10.29,30.23 10.79,30.73 11.56,30.73 12.32,29.97 12.95,29.97 14.48,28.45 18.29,28.45 v18.54,28.19
  Bottom 0.152: J10.6 1.32,24.31 | 2.92,26.04 2.92,30.1 2.54,30.48 2.54,31.45 v2.49,31.5 | v22.73,33.66 22.86,33.53 22.86,30.86 22.61,30.61 v22.61,27.3 22.48,27.43 20.45,27.43 19.94,27.94 19.94,28.32 19.68,28.57 18.92,28.57 v18.54,28.19
  Bottom 0.305: 1.32,24.31 1.32,24.43 2.92,26.04
PD2/D0/INT1  (via drill 0.25 pad 0.51)
  Top 0.152: J4.7 1.73,32.72 1.9,32.89 v1.9,33.27 1.86,33.32 J4.5 | J1.5 24.05,32.72 v23.75,33.02 24.05,33.32 J1.7 | J9.4 J9.3 | J5.1 J5.6 24.11,37.1 | U2.20 16.11,28.73 16.64,28.19 17.65,28.19 18.54,29.08 v18.85,29.08
  Route15 0.152: v1.9,33.27 2.29,32.89 3.94,32.89 6.22,30.61 9.14,30.61 10.29,31.75 17.65,31.75 18.29,32.38 19.05,32.38 | v23.75,33.02 23.5,33.02 22.73,32.26 19.18,32.26 19.05,32.38 | 19.05,32.38 v19.04,32.4
  Bottom 0.152: v23.75,33.02 23.75,33.66 23.11,34.29 23.11,36.07 23.37,36.32 | v18.85,29.08 18.67,29.08 18.29,29.46 18.29,30.35 19.43,31.5 19.43,32 v19.04,32.4 18.69,32.74 R26.1
  Bottom 0.305: v1.9,33.27 2.03,33.4 2.03,36.45 1.35,37.13 J9.4 | 23.37,36.32 23.88,36.83 23.88,36.86 J5.6
PD3/D1/INT2  (via drill 0.25 pad 0.51)
  Top 0.152: J9.5 J9.2 | J5.2 J5.5 24.11,39.39 | J4.6 4.44,33.02 5.33,33.91 v5.71,33.91 5.71,35.31 3.56,37.47 | U2.21 16.61,28.73 16.83,28.51 17.53,28.51 18.8,29.78 v18.86,29.78 | J1.6 v22.35,33.02
  Top 0.305: J9.5 1.59,39.43 3.56,37.47
  Route15 0.152: v5.71,33.91 6.73,32.89 20.07,32.89 v20.19,32.77 22.1,32.77 v22.35,33.02
  Bottom 0.152: 22.73,38.1 22.61,37.97 22.61,34.42 22.22,34.04 22.22,33.15 v22.35,33.02 | v20.19,32.77 20.17,32.74 R25.2 19.68,32.38 19.81,32.26 19.81,31.37 18.92,30.48 18.92,29.84 v18.86,29.78
  Bottom 0.305: J5.5 24.07,39.43 22.73,38.1
PF1/A4
  Top 0.152: U2.40 14.11,36.57 13.91,36.77 R13.1 C12.2 R16.2
VBAT  (via drill 0.25 pad 0.51)
  Top 0.305: J3.+ 19.05,37.72 19.56,38.23 19.56,39.37 19.18,39.75 15.75,39.75 14.55,38.55 C11.2 13.91,38.47 R13.2
  Bottom 0.203: TP1.T 17.42,36.32 17.52,36.42 | 17.52,36.42 17.67,36.56 | 17.52,36.42 17.75,36.42 17.78,36.45
  Bottom 0.305: U1.16 17.67,36.56 17.78,36.45 17.91,36.32 18.42,36.32 18.67,36.57 U1.14
  other vias: 19.68,36.32 19.05,36.2
  pour Bottom (isolate 0.254, no thermals): 20.07,36.52 20.07,35.58 19.54,35.05 18.16,35.05 18.03,35.18 18.03,36.2 18.54,36.7 19.89,36.7
  pour Top (isolate 0.254, no thermals): 19.94,35.94 18.67,35.94 18.42,36.2 18.42,38.35 18.54,38.48 19.81,38.48 20.07,38.23 20.07,36.07
VIN  (via drill 0.25 pad 0.51)
  Top 0.305: J4.2 3.12,34.22 v3.05,34.29 | J4.10 3.5,31.82 v3.18,31.5 | 21.41,34.22 J1.10 21.53,34.35 21.34,34.54 21.27,34.48 21.27,34.23 | J1.10 21.27,34.23 | 21.27,34.23 21.15,34.35 21.15,34.42 v21.34,34.61 | J1.2 21.84,31.82 | 21.84,31.82 21.9,31.82 21.97,31.75 | v21.97,31.37 21.97,31.69 21.84,31.82
  Top 0.508: J10.4 1.25,28.94 3.18,30.86 v3.18,31.5 | J10.4 J10.3 | J7.3 J7.4 21.97,31.09 v21.97,31.37 | R20.1 1.96,28.19 J10.4
  Route15 0.508: v3.05,34.29 3.3,34.54 9.02,34.54 10.16,33.4 20.57,33.4 21.34,34.16 v21.34,34.61
  Bottom 0.508: v3.18,31.5 3.18,34.16 v3.05,34.29 | v21.34,34.61 21.34,32 v21.97,31.37
VLED  (via drill 0.25 pad 0.51)
  Top 0.508: Q2.2 7.94,27.69 v7.43,28.19
  Top 0.61: Q2.2 8.38,27.69 Q1.3
  Bottom 0.305: C13.2 5.27,32.51
  Bottom 0.508: v7.43,28.19 7.43,29.15 F1.1 7.75,29.72 7.11,30.35 6.6,30.35 5.33,31.62 C14.2 5.27,32.51 5.27,33.04 U3.3
  other vias: 8.13,28.26
  pour Bottom (isolate 0.254, no thermals): 5.33,25.53 6.86,25.53 6.73,25.4 5.46,25.4
  pour Top (isolate 0.254, no thermals): 8.51,27.43 7.24,27.43 7.11,27.56 7.11,28.45 7.24,28.57 8.38,28.57 8.64,28.32 8.64,27.56
  pour Bottom (isolate 0.254, no thermals): 8.25,27.94 7.24,27.94 7.11,28.07 7.11,29.72 7.24,29.84 8.25,29.84 8.38,29.72 8.38,28.07
VSYS  (via drill 0.25 pad 0.51)
  Top 0.203: D1.+ 12.51,24.83 11.68,25.65 11.68,27.43 11.43,27.69 Q1.2
  Top 0.305: 7.93,29.91 U4.6 7.93,30.48 | 7.93,30.48 U4.1 7.93,32.7 7.77,32.87 R17.1 | D2.+ 8.22,30.52 | 8.19,30.52 7.97,30.52 7.93,30.48 | 8.22,30.52 7.95,30.79 | 8.22,30.52 8.19,30.52 | 8.19,30.52 7.95,30.28
  Top 0.61: Q1.2 10.54,27.69 9.91,28.32 9.91,29.69 9.59,30.01 | 9.59,30.01 D2.+ | 9.59,30.01 8.68,30.01 8.64,29.97
  Bottom 0.254: v16.51,37.34 16.51,37.72 16.65,37.86 U1.1 17.77,37.86 18.17,37.46 U1.15
  other vias: 16.95,37.02 12.45,37.27 12.38,37.85 7.87,37.47 7.24,37.47
  pour Bottom (isolate 0.254, no thermals): 6.73,38.48 6.73,37.37 7.01,37.08 13.97,37.08 14.22,37.34 14.22,38.48 13.97,38.73 6.99,38.73
  pour Route15 (isolate 0.254, no thermals): 11.56,37.08 12.45,37.08 13.33,36.2 17.02,36.2 17.27,36.45 17.27,37.29 17.09,37.47 13.97,37.47 13.33,38.1 11.56,38.1 11.43,37.97 11.43,37.21
  pour Top (no thermals): 9.4,33.66 9.4,30.18 8.31,29.08 7.75,29.08 7.62,29.21 7.62,33.15 6.86,33.91 6.86,37.59 6.99,37.72 8.13,37.72 8.25,37.59 8.25,34.8
VUSB  (via drill 0.25 pad 0.51)
  Top 0.305: U2.2 10.44,34.64 10.16,34.92 10.16,35.05 10.13,35.08 v10.16,35.12 | U2.7 10.15,32.14 v10.03,32.26
  Top 0.356: J2.1 9.94,38.2 10.29,37.85
  Bottom 0.254: U1.2 16.25,38.36 v16.13,38.48
  Bottom 0.305: R6.2 18.19,41.81 17.97,41.59 v17.97,41.02
  Bottom 0.508: 10.03,34.99 v10.16,35.12 10.41,34.86 10.41,34.54 | v10.03,32.26 10.41,32.64 10.41,34.16 | 10.41,34.16 10.41,34.54 | 10.41,34.54 9.91,35.05 | 10.41,34.54 10.92,35.05 | v22.16,39.5 22.16,39.24 C5.1 | 10.41,34.16 10.92,34.67
  other vias: 10.03,35.69 10.67,35.81 15.94,37.97
  pour Top (isolate 0.254, no thermals): 10.41,34.67 10.16,34.67 9.78,35.05 9.78,38.61 9.91,38.73 10.54,38.73 11.43,37.85 11.43,36.28 10.71,35.56 10.67,35.56 10.54,35.43 10.54,34.8
  pour Bottom (isolate 0.254, no thermals): 15.75,37.47 15.75,35.98 14.06,34.29 10.22,34.29 9.65,34.86 9.65,35.89 9.83,36.07 13.51,36.07 14.61,37.16 14.61,38.48 14.73,38.61 16.33,38.61 16.51,38.42 16.51,38.23
  pour Route15 (isolate 0.254, no thermals): 16.76,37.85 15.75,37.85 15.62,37.97 15.62,41.02 15.87,41.27 19.43,41.27 20.7,40 22.73,40 22.86,39.88 22.86,38.35 22.61,38.1 17.02,38.1

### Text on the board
tPlace: 6 | USB | BAT | 6 | 5 | 5 | 4 | - | + | 4 | 3 | 3 | 2 | 2 | 1 | MODE | 1
bPlace: GND | GND | INT2 | INT2 | INT1 | INT1 | Xadow Duino | 10/21/2015 | v1.0 | VCC | VCC | VLED | DO | GND | SCL | SCL | SDA | SDA
silk_top: - | +

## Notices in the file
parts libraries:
moudle-new: This work is licensed under the Creative Commons Attribution 4.0 International License.
To view a copy of this license,visit:
http://creativecommons.org/licenses/by-sa/4.0
moudle-new: CC-BY-SA
